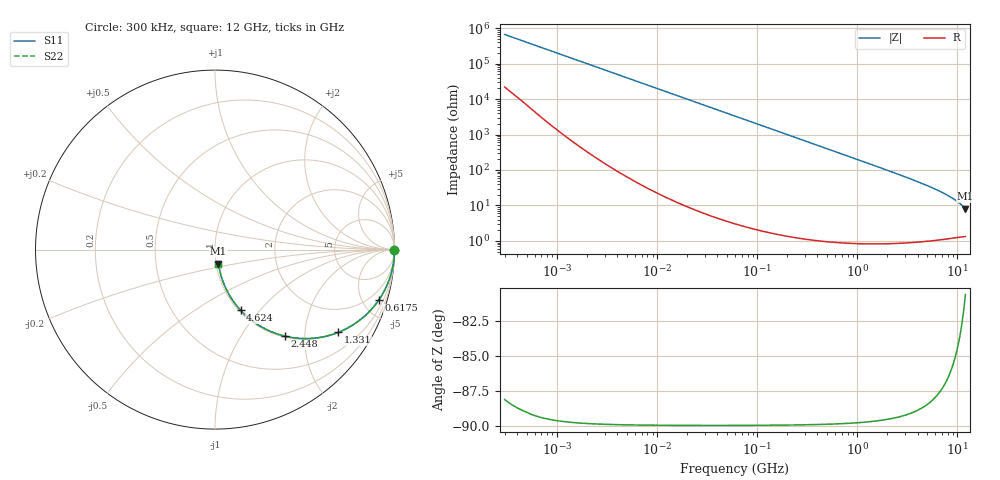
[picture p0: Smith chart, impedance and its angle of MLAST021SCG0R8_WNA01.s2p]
! MLAST021SCG0R8_WNA01  S-PARAMETER MODEL  ( General Type )
! Model Generated by TAIYO YUDEN Corporation (http://www.ty-top.com)
! Version 1.0
! TAIYO YUDEN Control No. 220901
! Copyright(c) 2022 TAIYO YUDEN CO.,LTD. All Rights Reserved.
! Product Description (link to TY-COMPAS)
! https://ds.yuden.co.jp/TYCOMPAS/or/detail?pn=MLAST021SCG0R8BWNA01&u=M
! Products Name : Multilayer Ceramic Capacitors
! Characteristics :
!  Capacitance : 0.8 pF , Rated Voltage : 25V , TCC : CG / C0G
!  Case Size : 0.25 x 0.125 / 0.0098 x 0.0049 [mm/inch] , Thickness : 0.125 / 0.0049 [mm/inch]
!  (Conditions: Temperature = 25 degC , DC Bias Current/Voltage = 0A / 0V)
! External Node Assignments :
!  1  o---| |---o  2
! GND o---------o GND
! Frequency Range : 0.3MHz  -  12000MHz  [ 401 STEP ]
# MHz S RI R 50
! Freq[MHz].  S11 Real  S11 Imag  S21 Real  S21 Imag  S12 Real  S12 Imag  S22 Real  S22 Imag
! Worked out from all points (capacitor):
!   401 points, 300 kHz to 12 GHz, reference 50 ohm
!   read as one part in series: C = 800 fF near 316.3 kHz
!   lowest |Z| = 8.17 ohm at 12 GHz (marker M1)
!   S11 on the Smith chart (normalised r, x): 300 kHz: open; 617.5 MHz: 1.02, -6.44; 1.331 GHz: 1.02, -2.97; 2.448 GHz: 1.02, -1.59; 4.624 GHz: 1.02, -0.79; 12 GHz: 1.03, -0.16
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0.3  1 -0.000151  5.01e-06 0.000151  5.01e-06 0.000151  1 -0.000151
0.316324  1 -0.000159  4.93e-06 0.000159  4.93e-06 0.000159  1 -0.000159
1.769972  1 -0.00089  4.06e-06 0.00089  4.06e-06 0.00089  1 -0.00089
10.44266  1 -0.00525  3.33e-05 0.00525  3.33e-05 0.00525  1 -0.00525
60  0.9991 -0.0301  0.000936 0.0301  0.000936 0.0301  0.9991 -0.0301
164.1901  0.9931 -0.082  0.00687 0.082  0.00687 0.082  0.9931 -0.082
244.3004  0.985 -0.121  0.015 0.121  0.015 0.121  0.985 -0.121
353.9943  0.969 -0.1724  0.031 0.1724  0.031 0.1724  0.969 -0.1724
473.7541  0.9458 -0.2253  0.0542 0.2253  0.0542 0.2253  0.9458 -0.2253
617.4538  0.9113 -0.283  0.0887 0.283  0.0887 0.283  0.9113 -0.283
918.7169  0.8224 -0.3802  0.1776 0.3802  0.1776 0.3802  0.8224 -0.3802
1331.232  0.6871 -0.4609  0.3129 0.4609  0.3129 0.4609  0.6871 -0.4609
1689.663  0.5754 -0.4907  0.4246 0.4907  0.4246 0.4907  0.5754 -0.4907
2088.533  0.4682 -0.4946  0.5318 0.4946  0.5318 0.4946  0.4682 -0.4946
2448.343  0.3886 -0.4821  0.6114 0.4821  0.6114 0.4821  0.3886 -0.4821
3364.605  0.247 -0.4235  0.753 0.4235  0.753 0.4235  0.247 -0.4235
4623.766  0.1424 -0.3376  0.8576 0.3376  0.8576 0.3376  0.1424 -0.3376
6188.031  0.0798 -0.2528  0.9202 0.2528  0.9202 0.2528  0.0798 -0.2528
8064.993  0.0448 -0.1789  0.9552 0.1789  0.9552 0.1789  0.0448 -0.1789
9708.23  0.0297 -0.1304  0.9703 0.1304  0.9703 0.1304  0.0297 -0.1304
11380.75  0.0213 -0.0909  0.9787 0.0909  0.9787 0.0909  0.0213 -0.0909
12000  0.0193 -0.0781  0.9807 0.0781  0.9807 0.0781  0.0193 -0.0781
